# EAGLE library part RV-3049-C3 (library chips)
The RV-3049-C3 is an ultra miniature Real-Time-Clock Module with embedded Crystal. This RTC has an SPI Bus (4-wire Serial- Interface) and offers temperature compensated time.
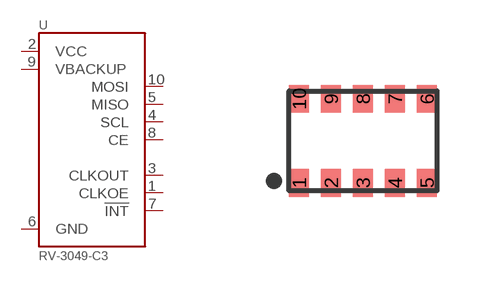
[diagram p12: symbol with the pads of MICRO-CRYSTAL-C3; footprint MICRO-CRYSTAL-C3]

Designator prefix U

## RV-3049-C3  [MICRO-CRYSTAL-C3]
1  CLKOE
2  VCC
3  CLKOUT
4  SCL
5  MISO
6  GND
7  !INT
8  CE
9  VBACKUP
10  MOSI

## Footprint MICRO-CRYSTAL-C3 (pad centres in mm)
smd 0.5 x 0.7: 1 -1.6,-1.05; 2 -0.8,-1.05; 3 0,-1.05; 4 0.8,-1.05; 5 1.6,-1.05; 6 1.6,1.05; 7 0.8,1.05; 8 0,1.05; 9 -0.8,1.05; 10 -1.6,1.05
